| IBIS file stm32f7x3_wlcsp100.ibs
[IBIS ver] 4.2
[File name] stm32f7x3_wlcsp100.ibs
[File Rev] 1.1
[Date]  21-12-2016
[Source] Data Created at STMicroelectronics
[Notes]  File originated from ELDO simulations.
[Disclaimer]  This information is for modeling purpose only and is
   not guaranted.
   The information is subject to change without notice.
[Copyright] Copyright 2017 STMicroelectronics Inc.
|   Component stm32f7x3_wlcsp100
[Component] stm32f7x3_wlcsp100
[Manufacturer] STMicroelectronics
[Package]
| variable   typ   min   max
R_pkg   0.0   0.0   0.0
L_pkg   0.0H   0.0H   0.0H
C_pkg   0.0F   0.0F   0.0F
[Pin]  signal_name   model_name   R_pin   L_pin   C_pin
A1 VDD power
A10 PE3 io8p_arsudq_ft
A2 VSS gnd
A3 PC10 io8p_arsudq_ft
A4 PD1 io8p_arsudq_ft
A5 PD5 io8p_arsudq_ft
A6 PB3 io8p_arsudq_ft
A7 BOOT0 vpp_test_hv
A8 VSS gnd
A9 VDD power
B1 PA13 io8p_arsudq_ft
B10 PE6 io8p_arsudq_ft
B2 PA12 io8usb_lsfs_otg_ft
B3 VCAP_2 power
B4 PA15 io8p_arsudq_ft
B5 PD0 io8p_arsudq_ft
B6 PD4 io8p_arsudq_ft
B7 PB4 io8p_arsudq_ft
B8 PB7 io8p_arsudq_i2c_ft
B9 PE1 io8p_arsudq_ft
C1 PA11 io8usb_lsfs_otg_ft
C10 VBAT power
C2 PA10 io8usb_id_otg_ft
C3 PA9 io8usb_vbus_otg_ft
C4 PA14 io8p_arsudq_ft
C5 PC11 io8p_arsudq_ft
C6 PD3 io8p_arsudq_ft
C7 PB5 io8p_ar3wsudq_ft
C8 PB8 io8p_arsudq_i2c_ft
C9 PE2 io8p_arsudq_ft
D1 PC9 io8p_arsudq_i2c_ft
D10 PC13 io8p_arwsudq_ft_v33
D2 PC8 io8p_arsudq_ft
D3 PA8 io8p_arsudq_i2c_ft
D4 PC7 io8p_arsudq_ft
D5 PC12 io8p_arsudq_ft
D6 PD6 io8p_arsudq_ft
D7 PB6 io8p_arsudq_i2c_ft
D8 PB9 io8p_arsudq_i2c_ft
D9 PE4 io8p_arsudq_ft
E1 PC6 io8p_arsudq_ft
E10 PC15-OSC32_OUT io8p_arwsudq_ft
E2 PD15 io8p_arsudq_ft
E3 PD13 io8p_arsudq_ft
E4 PE10 io8p_arsudq_ft
E5 PD2 io8p_arsudq_ft
E6 PD7 io8p_arsudq_ft
E7 PE0 io8p_arsudq_ft
E8 PE5 io8p_arsudq_ft
E9 PC14-OSC32_IN io8p_arwsudq_ft_v33
F1 PD14 io8p_arsudq_ft
F10 VDD power
F2 PD12 io8p_arsudq_ft
F3 PD11 io8p_arsudq_ft
F4 PE15 io8p_ar3wsudq_ft
F5 PB0 io8p_ar3wsudq_ft
F6 PA5 io8p_ar3wsudq_ft
F7 PC3 io8p_ar3wsudq_ft
F8 PC0 io8p_ar3wsudq_ft
F9 VSS power
G1 VDD12OTGHS power
G10 PH0-OSC_IN io8p_arsudq_ft
G2 OTG_HS_REXT gnd
G3 PB10 io8p_arsudq_i2c_ft
G4 PE11 io8p_arsudq_ft
G5 PB1 io8p_ar3wsudq_ft
G6 PA6 io8p_ar3wsudq_ft
G7 PA4 io8p_ar3wsudq_ft
G8 PA0-WKUP io8p_ar3wsudq_ft_v33
G9 NRST ioreset_ft_v33
H1 PB15 io8p_arsudq_ft
H10 PH1-OSC_OUT io8p_arsudq_ft
H2 PB13 io8usb_vbus_otg_ft
H3 PB11 io8p_arsudq_i2c_ft
H4 PE12 io8p_arsudq_ft
H5 PE8 io8p_arsudq_ft
H6 PC4 io8p_ar3wsudq_ft
H7 PA3 io8p_ar3wsudq_ft
H8 PA2 io8p_ar3wsudq_ft_v33
H9 PC1 io8p_ar3wsudq_ft_v33
J1 PB14 io8p_arsudq_ft
J10 PC2 io8p_ar3wsudq_ft
J2 PB12 io8usb_id_otg_ft
J3 VCAP_1 power
J4 PE13 io8p_arsudq_ft
J5 PE7 io8p_arsudq_ft
J6 PC5 io8p_ar3wsudq_ft
J7 VDD power
J8 PA1 io8p_ar3wsudq_ft
J9 VREF+ power
K1 VDDUSB power
K10 VSSA gnd
K2 VDD power
K3 VSS gnd
K4 PE14 io8p_arsudq_ft
K5 PE9 io8p_arsudq_ft
K6 PB2 io8p_ar3wsudq_ft
K7 PA7 io8p_ar3wsudq_ft
K8 VSS gnd
K9 VDDA power
[Diff Pin]   inv_pin   vdiff   tdelay_typ  tdelay_min  tdelay_max
B2   C1   200mV   NA   NA   NA
[Model Selector] io8p_ar3wsudq_ft
io8p00_ar3wsudq_ft_pd_lv  "SPEED00 1P8V, PD=40kOhm"
io8p00_ar3wsudq_ft_pu_lv  "SPEED00 1P8V, PU=40kOhm"
io8p00_ar3wsudq_ft_lv  "SPEED00 1P8V"
io8p01_ar3wsudq_ft_pd_lv  "SPEED01 1P8V, PD=40kOhm"
io8p01_ar3wsudq_ft_pu_lv  "SPEED01 1P8V, PU=40kOhm"
io8p01_ar3wsudq_ft_lv  "SPEED01 1P8V"
io8p10_ar3wsudq_ft_pd_lv  "SPEED10 1P8V, PD=40kOhm"
io8p10_ar3wsudq_ft_pu_lv  "SPEED10 1P8V, PU=40kOhm"
io8p10_ar3wsudq_ft_lv  "SPEED10 1P8V"
io8p11_ar3wsudq_ft_pd_lv  "SPEED11 1P8V, PD=40kOhm"
io8p11_ar3wsudq_ft_pu_lv  "SPEED11 1P8V, PU=40kOhm"
io8p11_ar3wsudq_ft_lv  "SPEED11 1P8V"
io8p00_ar3wsudq_ft_pd  "SPEED00, PD=40kOhm"
io8p00_ar3wsudq_ft_pu  "SPEED00, PU=40kOhm"
io8p00_ar3wsudq_ft  "SPEED00"
io8p01_ar3wsudq_ft_pd  "SPEED01, PD=40kOhm"
io8p01_ar3wsudq_ft_pu  "SPEED01, PU=40kOhm"
io8p01_ar3wsudq_ft  "SPEED01"
io8p10_ar3wsudq_ft_pd  "SPEED10, PD=40kOhm"
io8p10_ar3wsudq_ft_pu  "SPEED10, PU=40kOhm"
io8p10_ar3wsudq_ft  "SPEED10"
io8p11_ar3wsudq_ft_pd  "SPEED11, PD=40kOhm"
io8p11_ar3wsudq_ft_pu  "SPEED11, PU=40kOhm"
io8p11_ar3wsudq_ft  "SPEED11"
[Model Selector] io8p_ar3wsudq_ft_v33
io8p00_ar3wsudq_ft_v33_pd_lv  "SPEED00 1P8V, PD=40kOhm"
io8p00_ar3wsudq_ft_v33_pu_lv  "SPEED00 1P8V, PU=40kOhm"
io8p00_ar3wsudq_ft_v33_lv  "SPEED00 1P8V"
io8p01_ar3wsudq_ft_v33_pd_lv  "SPEED01 1P8V, PD=40kOhm"
io8p01_ar3wsudq_ft_v33_pu_lv  "SPEED01 1P8V, PU=40kOhm"
io8p01_ar3wsudq_ft_v33_lv  "SPEED01 1P8V"
io8p10_ar3wsudq_ft_v33_pd_lv  "SPEED10 1P8V, PD=40kOhm"
io8p10_ar3wsudq_ft_v33_pu_lv  "SPEED10 1P8V, PU=40kOhm"
io8p10_ar3wsudq_ft_v33_lv  "SPEED10 1P8V"
io8p11_ar3wsudq_ft_v33_pd_lv  "SPEED11 1P8V, PD=40kOhm"
io8p11_ar3wsudq_ft_v33_pu_lv  "SPEED11 1P8V, PU=40kOhm"
io8p11_ar3wsudq_ft_v33_lv  "SPEED11 1P8V"
io8p00_ar3wsudq_ft_v33_pd  "SPEED00, PD=40kOhm"
io8p00_ar3wsudq_ft_v33_pu  "SPEED00, PU=40kOhm"
io8p00_ar3wsudq_ft_v33  "SPEED00"
io8p01_ar3wsudq_ft_v33_pd  "SPEED01, PD=40kOhm"
io8p01_ar3wsudq_ft_v33_pu  "SPEED01, PU=40kOhm"
io8p01_ar3wsudq_ft_v33  "SPEED01"
io8p10_ar3wsudq_ft_v33_pd  "SPEED10, PD=40kOhm"
io8p10_ar3wsudq_ft_v33_pu  "SPEED10, PU=40kOhm"
io8p10_ar3wsudq_ft_v33  "SPEED10"
io8p11_ar3wsudq_ft_v33_pd  "SPEED11, PD=40kOhm"
io8p11_ar3wsudq_ft_v33_pu  "SPEED11, PU=40kOhm"
io8p11_ar3wsudq_ft_v33  "SPEED11"
[Model Selector] io8p_arsudq_ft
io8p00_arsudq_ft_pd_lv  "SPEED00 1P8V, PD=40kOhm"
io8p00_arsudq_ft_pu_lv  "SPEED00 1P8V, PU=40kOhm"
io8p00_arsudq_ft_lv  "SPEED00 1P8V"
io8p01_arsudq_ft_pd_lv  "SPEED01 1P8V, PD=40kOhm"
io8p01_arsudq_ft_pu_lv  "SPEED01 1P8V, PU=40kOhm"
io8p01_arsudq_ft_lv  "SPEED01 1P8V"
io8p10_arsudq_ft_pd_lv  "SPEED10 1P8V, PD=40kOhm"
io8p10_arsudq_ft_pu_lv  "SPEED10 1P8V, PU=40kOhm"
io8p10_arsudq_ft_lv  "SPEED10 1P8V"
io8p11_arsudq_ft_pd_lv  "SPEED11 1P8V, PD=40kOhm"
io8p11_arsudq_ft_pu_lv  "SPEED11 1P8V, PU=40kOhm"
io8p11_arsudq_ft_lv  "SPEED11 1P8V"
io8p00_arsudq_ft_pd  "SPEED00, PD=40kOhm"
io8p00_arsudq_ft_pu  "SPEED00, PU=40kOhm"
io8p00_arsudq_ft  "SPEED00"
io8p01_arsudq_ft_pd  "SPEED01, PD=40kOhm"
io8p01_arsudq_ft_pu  "SPEED01, PU=40kOhm"
io8p01_arsudq_ft  "SPEED01"
io8p10_arsudq_ft_pd  "SPEED10, PD=40kOhm"
io8p10_arsudq_ft_pu  "SPEED10, PU=40kOhm"
io8p10_arsudq_ft  "SPEED10"
io8p11_arsudq_ft_pd  "SPEED11, PD=40kOhm"
io8p11_arsudq_ft_pu  "SPEED11, PU=40kOhm"
io8p11_arsudq_ft  "SPEED11"
[Model Selector] io8p_arsudq_i2c_ft
io8prog_1v8_i2c_pd  "5V Tol GPIO 1.8V range i2c functionality with pull down"
io8prog_1v8_i2c_pu  "5V Tol GPIO 1.8V range i2c functionality with pull up"
io8prog_1v8_i2c  "5V Tol GPIO 1.8V range i2c functionality"
io8prog_3v3_i2c_pd  "5V Tol GPIO 3.3V range i2c functionality with pull down"
io8prog_3v3_i2c_pu  "5V Tol GPIO 3.3V range i2c functionality with pull up"
io8prog_3v3_i2c  "5V Tol GPIO 3.3V range i2c functionality"
io8prog_1v8_pd_00  "5V Tol GPIO 1.8V range with pd speed 00"
io8prog_1v8_pu_00  "5V Tol GPIO 1.8V range with pu speed 00"
io8prog_1v8_00  "5V Tol GPIO 1.8V range speed 00"
io8prog_3v3_pd_00  "5V Tol GPIO 3.3V range with pd speed 00"
io8prog_3v3_pu_00  "5V Tol GPIO 3.3V range with pu speed 00"
io8prog_3v3_00  "5V Tol GPIO 3.3V range speed 00"
io8prog_1v8_pd_01  "5V Tol GPIO 1.8V range with pd speed 01"
io8prog_1v8_pu_01  "5V Tol GPIO 1.8V range with pu speed 01"
io8prog_1v8_01  "5V Tol GPIO 1.8V range speed 01"
io8prog_3v3_pd_01  "5V Tol GPIO 3.3V range with pd speed 01"
io8prog_3v3_pu_01  "5V Tol GPIO 3.3V range with pu speed 01"
io8prog_3v3_01  "5V Tol GPIO 3.3V range speed 01"
io8prog_1v8_pd_10  "5V Tol GPIO 1.8V range with pd speed 10"
io8prog_1v8_pu_10  "5V Tol GPIO 1.8V range with pu speed 10"
io8prog_1v8_10  "5V Tol GPIO 1.8V range speed 10"
io8prog_3v3_pd_10  "5V Tol GPIO 3.3V range with pd speed 10"
io8prog_3v3_pu_10  "5V Tol GPIO 3.3V range with pu speed 10"
io8prog_3v3_10  "5V Tol GPIO 3.3V range speed 10"
io8prog_1v8_pd_11  "5V Tol GPIO 1.8V range with pd speed 11"
io8prog_1v8_pu_11  "5V Tol GPIO 1.8V range with pu speed 11"
io8prog_1v8_11  "5V Tol GPIO 1.8V range speed 11"
io8prog_3v3_pd_11  "5V Tol GPIO 3.3V range with pd speed 11"
io8prog_3v3_pu_11  "5V Tol GPIO 3.3V range with pu speed 11"
io8prog_3v3_11  "5V Tol GPIO 3.3V range speed 11"
[Model Selector] io8p_arwsudq_ft
io8p00_arwsudq_ft_pd_lv  "SPEED00 1P8V, PD=40kOhm"
io8p00_arwsudq_ft_pu_lv  "SPEED00 1P8V, PU=40kOhm"
io8p00_arwsudq_ft_lv  "SPEED00 1P8V"
io8p01_arwsudq_ft_pd_lv  "SPEED01 1P8V, PD=40kOhm"
io8p01_arwsudq_ft_pu_lv  "SPEED01 1P8V, PU=40kOhm"
io8p01_arwsudq_ft_lv  "SPEED01 1P8V"
io8p10_arwsudq_ft_pd_lv  "SPEED10 1P8V, PD=40kOhm"
io8p10_arwsudq_ft_pu_lv  "SPEED10 1P8V, PU=40kOhm"
io8p10_arwsudq_ft_lv  "SPEED10 1P8V"
io8p11_arwsudq_ft_pd_lv  "SPEED11 1P8V, PD=40kOhm"
io8p11_arwsudq_ft_pu_lv  "SPEED11 1P8V, PU=40kOhm"
io8p11_arwsudq_ft_lv  "SPEED11 1P8V"
io8p00_arwsudq_ft_pd  "SPEED00, PD=40kOhm"
io8p00_arwsudq_ft_pu  "SPEED00, PU=40kOhm"
io8p00_arwsudq_ft  "SPEED00"
io8p01_arwsudq_ft_pd  "SPEED01, PD=40kOhm"
io8p01_arwsudq_ft_pu  "SPEED01, PU=40kOhm"
io8p01_arwsudq_ft  "SPEED01"
io8p10_arwsudq_ft_pd  "SPEED10, PD=40kOhm"
io8p10_arwsudq_ft_pu  "SPEED10, PU=40kOhm"
io8p10_arwsudq_ft  "SPEED10"
io8p11_arwsudq_ft_pd  "SPEED11, PD=40kOhm"
io8p11_arwsudq_ft_pu  "SPEED11, PU=40kOhm"
io8p11_arwsudq_ft  "SPEED11"
[Model Selector] io8p_arwsudq_ft_v33
io8p00_arwsudq_ft_v33_pd_lv  "SPEED00 1P8V, PD=40kOhm"
io8p00_arwsudq_ft_v33_pu_lv  "SPEED00 1P8V, PU=40kOhm"
io8p00_arwsudq_ft_v33_lv  "SPEED00 1P8V"
io8p01_arwsudq_ft_v33_pd_lv  "SPEED01 1P8V, PD=40kOhm"
io8p01_arwsudq_ft_v33_pu_lv  "SPEED01 1P8V, PU=40kOhm"
io8p01_arwsudq_ft_v33_lv  "SPEED01 1P8V"
io8p10_arwsudq_ft_v33_pd_lv  "SPEED10 1P8V, PD=40kOhm"
io8p10_arwsudq_ft_v33_pu_lv  "SPEED10 1P8V, PU=40kOhm"
io8p10_arwsudq_ft_v33_lv  "SPEED10 1P8V"
io8p11_arwsudq_ft_v33_pd_lv  "SPEED11 1P8V, PD=40kOhm"
io8p11_arwsudq_ft_v33_pu_lv  "SPEED11 1P8V, PU=40kOhm"
io8p11_arwsudq_ft_v33_lv  "SPEED11 1P8V"
io8p00_arwsudq_ft_v33_pd  "SPEED00, PD=40kOhm"
io8p00_arwsudq_ft_v33_pu  "SPEED00, PU=40kOhm"
io8p00_arwsudq_ft_v33  "SPEED00"
io8p01_arwsudq_ft_v33_pd  "SPEED01, PD=40kOhm"
io8p01_arwsudq_ft_v33_pu  "SPEED01, PU=40kOhm"
io8p01_arwsudq_ft_v33  "SPEED01"
io8p10_arwsudq_ft_v33_pd  "SPEED10, PD=40kOhm"
io8p10_arwsudq_ft_v33_pu  "SPEED10, PU=40kOhm"
io8p10_arwsudq_ft_v33  "SPEED10"
io8p11_arwsudq_ft_v33_pd  "SPEED11, PD=40kOhm"
io8p11_arwsudq_ft_v33_pu  "SPEED11, PU=40kOhm"
io8p11_arwsudq_ft_v33  "SPEED11"
[Model Selector] io8usb_id_otg_ft
io8p00_id_otg_ft_pd_lv  "SPEED00 1P8V, PD=14kOhm"
io8p00_id_otg_ft_pu_lv  "SPEED00 1P8V, PU=14kOhm"
io8p00_id_otg_ft_lv  "SPEED00 1P8V"
io8p01_id_otg_ft_pd_lv  "SPEED01 1P8V, PD=14kOhm"
io8p01_id_otg_ft_pu_lv  "SPEED01 1P8V, PU=14kOhm"
io8p01_id_otg_ft_lv  "SPEED01 1P8V"
io8p10_id_otg_ft_pd_lv  "SPEED10 1P8V, PD=14kOhm"
io8p10_id_otg_ft_pu_lv  "SPEED10 1P8V, PU=14kOhm"
io8p10_id_otg_ft_lv  "SPEED10 1P8V"
io8p11_id_otg_ft_pd_lv  "SPEED11 1P8V, PD=14kOhm"
io8p11_id_otg_ft_pu_lv  "SPEED11 1P8V, PU=14kOhm"
io8p11_id_otg_ft_lv  "SPEED11 1P8V"
io8p00_id_otg_ft_pd  "SPEED00, PD=14kOhm"
io8p00_id_otg_ft_pu  "SPEED00, PU=14kOhm"
io8p00_id_otg_ft  "SPEED00"
io8p01_id_otg_ft_pd  "SPEED01, PD=14kOhm"
io8p01_id_otg_ft_pu  "SPEED01, PU=14kOhm"
io8p01_id_otg_ft  "SPEED01"
io8p10_id_otg_ft_pd  "SPEED10, PD=14kOhm"
io8p10_id_otg_ft_pu  "SPEED10, PU=14kOhm"
io8p10_id_otg_ft  "SPEED10"
io8p11_id_otg_ft_pd  "SPEED11, PD=14kOhm"
io8p11_id_otg_ft_pu  "SPEED11, PU=14kOhm"
io8p11_id_otg_ft  "SPEED11"
[Model Selector] io8usb_lsfs_otg_ft
io8usb_ls_otg_ft_dpdn_pd  "LS USB DP/DN IO + PD=20kOhm"
io8usb_ls_otg_ft_dpdn_pupu2  "LS USB DP/DN IO + PU/PU2=2.2kOhm"
io8usb_ls_otg_ft_dpdn_pu2  "LS USB DP/DN IO + PU2=1.2kOhm"
io8usb_ls_otg_ft_dpdn_pu  "LS USB DP/DN IO + PU=1.2kOhm"
io8usb_ls_otg_ft_dpdn  "LS USB DP/DN IO"
io8usb_fs_otg_ft_dpdn_pd  "HS USB DP/DN IO + PD=20kOhm"
io8usb_fs_otg_ft_dpdn_pupu2  "HS USB DP/DN IO + PU/PU2=2.2kOhm"
io8usb_fs_otg_ft_dpdn_pu2  "HS USB DP/DN IO + PU2=1.2kOhm"
io8usb_fs_otg_ft_dpdn_pu  "HS USB DP/DN IO + PU=1.2kOhm"
io8usb_fs_otg_ft_dpdn  "HS USB DP/DN IO"
io8p00_lsfs_otg_ft_pd_lv  "SPEED00 1P8V, PD=40kOhm"
io8p00_lsfs_otg_ft_pu_lv  "SPEED00 1P8V, PU=40kOhm"
io8p00_lsfs_otg_ft_lv  "SPEED00 1P8V"
io8p01_lsfs_otg_ft_pd_lv  "SPEED01 1P8V, PD=40kOhm"
io8p01_lsfs_otg_ft_pu_lv  "SPEED01 1P8V, PU=40kOhm"
io8p01_lsfs_otg_ft_lv  "SPEED01 1P8V"
io8p10_lsfs_otg_ft_pd_lv  "SPEED10 1P8V, PD=40kOhm"
io8p10_lsfs_otg_ft_pu_lv  "SPEED10 1P8V, PU=40kOhm"
io8p10_lsfs_otg_ft_lv  "SPEED10 1P8V"
io8p11_lsfs_otg_ft_pd_lv  "SPEED11 1P8V, PD=40kOhm"
io8p11_lsfs_otg_ft_pu_lv  "SPEED11 1P8V, PU=40kOhm"
io8p11_lsfs_otg_ft_lv  "SPEED11 1P8V"
io8p00_lsfs_otg_ft_pd  "SPEED00, PD=40kOhm"
io8p00_lsfs_otg_ft_pu  "SPEED00, PU=40kOhm"
io8p00_lsfs_otg_ft  "SPEED00"
io8p01_lsfs_otg_ft_pd  "SPEED01, PD=40kOhm"
io8p01_lsfs_otg_ft_pu  "SPEED01, PU=40kOhm"
io8p01_lsfs_otg_ft  "SPEED01"
io8p10_lsfs_otg_ft_pd  "SPEED10, PD=40kOhm"
io8p10_lsfs_otg_ft_pu  "SPEED10, PU=40kOhm"
io8p10_lsfs_otg_ft  "SPEED10"
io8p11_lsfs_otg_ft_pd  "SPEED11, PD=40kOhm"
io8p11_lsfs_otg_ft_pu  "SPEED11, PU=40kOhm"
io8p11_lsfs_otg_ft  "SPEED11"
[Model Selector] io8usb_vbus_otg_ft
io8psenb_vbus_otg_ft  "VBUS PULSE, SENSE VB"
io8psenab_vbus_otg_ft  "VBUS PULSE, SENSE VA and VB"
io8psena_vbus_otg_ft  "VBUS PULSE, SENSE VA"
io8psen_vbus_otg_ft  "VBUS PULSE"
io8p00_vbus_otg_ft_pd_lv  "SPEED00 1P8V, PD=40kOhm"
io8p00_vbus_otg_ft_pu_lv  "SPEED00 1P8V, PU=40kOhm"
io8p00_vbus_otg_ft_lv  "SPEED00 1P8V"
io8p01_vbus_otg_ft_pd_lv  "SPEED01 1P8V, PD=40kOhm"
io8p01_vbus_otg_ft_pu_lv  "SPEED01 1P8V, PU=40kOhm"
io8p01_vbus_otg_ft_lv  "SPEED01 1P8V"
io8p10_vbus_otg_ft_pd_lv  "SPEED10 1P8V, PD=40kOhm"
io8p10_vbus_otg_ft_pu_lv  "SPEED10 1P8V, PU=40kOhm"
io8p10_vbus_otg_ft_lv  "SPEED10 1P8V"
io8p11_vbus_otg_ft_pd_lv  "SPEED11 1P8V, PD=40kOhm"
io8p11_vbus_otg_ft_pu_lv  "SPEED11 1P8V, PU=40kOhm"
io8p11_vbus_otg_ft_lv  "SPEED11 1P8V"
io8p00_vbus_otg_ft_pd  "SPEED00, PD=40kOhm"
io8p00_vbus_otg_ft_pu  "SPEED00, PU=40kOhm"
io8p00_vbus_otg_ft  "SPEED00"
io8p01_vbus_otg_ft_pd  "SPEED01, PD=40kOhm"
io8p01_vbus_otg_ft_pu  "SPEED01, PU=40kOhm"
io8p01_vbus_otg_ft  "SPEED01"
io8p10_vbus_otg_ft_pd  "SPEED10, PD=40kOhm"
io8p10_vbus_otg_ft_pu  "SPEED10, PU=40kOhm"
io8p10_vbus_otg_ft  "SPEED10"
io8p11_vbus_otg_ft_pd  "SPEED11, PD=40kOhm"
io8p11_vbus_otg_ft_pu  "SPEED11, PU=40kOhm"
io8p11_vbus_otg_ft  "SPEED11"
[Model Selector] ioreset_ft_v33
ioreset_ft_v33_pu_lv  "IORESET 1P8V + PU=40kOhm"
ioreset_ft_v33_nopu_lv  "IORESET 1P8V"
ioreset_ft_v33_pu  "IORESET + PU=40kOhm"
ioreset_ft_v33_nopu  "IORESET"
[Model Selector] vpp_test_hv
vpp_test_hv_2p4  "Input Buffer 1P8V"
vpp_test_hv_3p3  "Input Buffer"
| Models and submodels in the file (242): io8p00_ar3wsudq_ft_pd_lv (I/O), io8p00_ar3wsudq_ft_pu_lv (I/O), io8p00_ar3wsudq_ft_lv (I/O), io8p01_ar3wsudq_ft_pd_lv (I/O), io8p01_ar3wsudq_ft_pu_lv (I/O), io8p01_ar3wsudq_ft_lv (I/O), io8p10_ar3wsudq_ft_pd_lv (I/O), io8p10_ar3wsudq_ft_pu_lv (I/O), io8p10_ar3wsudq_ft_lv (I/O), io8p11_ar3wsudq_ft_pd_lv (I/O), io8p11_ar3wsudq_ft_pu_lv (I/O), io8p11_ar3wsudq_ft_lv (I/O), io8p00_ar3wsudq_ft_pd (I/O), io8p00_ar3wsudq_ft_pu (I/O), io8p00_ar3wsudq_ft (I/O), io8p01_ar3wsudq_ft_pd (I/O), io8p01_ar3wsudq_ft_pu (I/O), io8p01_ar3wsudq_ft (I/O), io8p10_ar3wsudq_ft_pd (I/O), io8p10_ar3wsudq_ft_pu (I/O), io8p10_ar3wsudq_ft (I/O), io8p11_ar3wsudq_ft_pd (I/O), io8p11_ar3wsudq_ft_pu (I/O), io8p11_ar3wsudq_ft (I/O), io8p00_ar3wsudq_ft_v33_pd_lv (I/O), io8p00_ar3wsudq_ft_v33_pu_lv (I/O), io8p00_ar3wsudq_ft_v33_lv (I/O), io8p01_ar3wsudq_ft_v33_pd_lv (I/O), io8p01_ar3wsudq_ft_v33_pu_lv (I/O), io8p01_ar3wsudq_ft_v33_lv (I/O), io8p10_ar3wsudq_ft_v33_pd_lv (I/O), io8p10_ar3wsudq_ft_v33_pu_lv (I/O), io8p10_ar3wsudq_ft_v33_lv (I/O), io8p11_ar3wsudq_ft_v33_pd_lv (I/O), io8p11_ar3wsudq_ft_v33_pu_lv (I/O), io8p11_ar3wsudq_ft_v33_lv (I/O), io8p00_ar3wsudq_ft_v33_pd (I/O), io8p00_ar3wsudq_ft_v33_pu (I/O), io8p00_ar3wsudq_ft_v33 (I/O), io8p01_ar3wsudq_ft_v33_pd (I/O), io8p01_ar3wsudq_ft_v33_pu (I/O), io8p01_ar3wsudq_ft_v33 (I/O), io8p10_ar3wsudq_ft_v33_pd (I/O), io8p10_ar3wsudq_ft_v33_pu (I/O), io8p10_ar3wsudq_ft_v33 (I/O), io8p11_ar3wsudq_ft_v33_pd (I/O), io8p11_ar3wsudq_ft_v33_pu (I/O), io8p11_ar3wsudq_ft_v33 (I/O), io8p00_arsudq_ft_pd_lv (I/O), io8p00_arsudq_ft_pu_lv (I/O), io8p00_arsudq_ft_lv (I/O), io8p01_arsudq_ft_pd_lv (I/O), io8p01_arsudq_ft_pu_lv (I/O), io8p01_arsudq_ft_lv (I/O), io8p10_arsudq_ft_pd_lv (I/O), io8p10_arsudq_ft_pu_lv (I/O), io8p10_arsudq_ft_lv (I/O), io8p11_arsudq_ft_pd_lv (I/O), io8p11_arsudq_ft_pu_lv (I/O), io8p11_arsudq_ft_lv (I/O), io8p00_arsudq_ft_pd (I/O), io8p00_arsudq_ft_pu (I/O), io8p00_arsudq_ft (I/O), io8p01_arsudq_ft_pd (I/O), io8p01_arsudq_ft_pu (I/O), io8p01_arsudq_ft (I/O), io8p10_arsudq_ft_pd (I/O), io8p10_arsudq_ft_pu (I/O), io8p10_arsudq_ft (I/O), io8p11_arsudq_ft_pd (I/O), io8p11_arsudq_ft_pu (I/O), io8p11_arsudq_ft (I/O), io8prog_1v8_i2c_pd (I/O), io8prog_1v8_i2c_pu (I/O), io8prog_1v8_i2c (I/O), io8prog_3v3_i2c_pd (I/O), io8prog_3v3_i2c_pu (I/O), io8prog_3v3_i2c (I/O), io8prog_1v8_pd_00 (I/O), io8prog_1v8_pu_00 (I/O)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
